VAR_GLOBAL
	

	nullInputChannel : NullDigitalInputChannel;
	
	device1 : EL1008;
	
	myFanControlDigitalInput : AssignableDigitalInputChannel(nullInputChannel);
	
	myFanControl : TwoStateSwitch(myFanControlDigitalInput);

END_VAR
